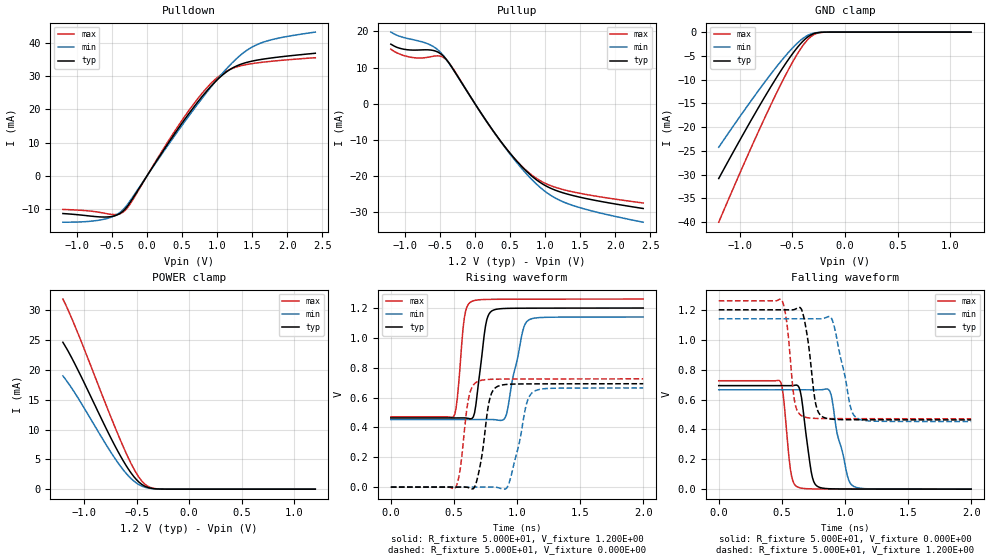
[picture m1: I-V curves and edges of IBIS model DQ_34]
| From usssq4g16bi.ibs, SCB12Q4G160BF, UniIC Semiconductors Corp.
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|   Model DQ_34
[Model] DQ_34
Model_type I/O
Polarity   Non-Inverting
Enable   Active-High
Vinl =  8.300E-01
Vinh =  9.700E-01
Vmeas =  8.400E-01
Rref =  5.000E+01
Vref =  1.200E+00
C_comp   7.488E-13   7.319E-13   7.703E-13
C_comp_pullup   2.702E-13   2.654E-13   2.792E-13
C_comp_pulldown   4.786E-13   4.665E-13   4.911E-13
[Model Spec]
Vinh   9.700E-01   9.250E-01   1.015E+00
Vinl   8.300E-01   7.850E-01   8.750E-01
Vmeas   8.400E-01   7.980E-01   8.820E-01
Vref   1.200E+00   1.140E+00   1.260E+00
Rref   5.000E+01   5.000E+01   5.000E+01
[Temperature Range]   45.000   95.000   -40.000
[Voltage Range]   1.200E+00   1.140E+00   1.260E+00
[C Comp Corner]
C_comp_pullup   2.702E-13   2.654E-13   2.792E-13
C_comp_pulldown   4.786E-13   4.665E-13   4.911E-13
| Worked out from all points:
|   slope of the pulldown table from 0 to 0.18 V, typ, clamps not added: 30.5 ohm
|   slope of the pullup table from 0 to 0.18 V, typ, clamps not added: 34 ohm
|   GND clamp passes 1 mA (typ) near -0.35 V on its own axis
|   POWER clamp passes 1 mA (typ) near -0.46 V on its own axis
|   rising waveform, R_fixture 5.000E+01, V_fixture 1.200E+00: 20-80 % time 63.1ps typ, 95.3ps min, 47.4ps max; typ from 0.463 V to 1.2 V
|   rising waveform, R_fixture 5.000E+01, V_fixture 0.000E+00: 20-80 % time 68.5ps typ, 98.1ps min, 59ps max; typ from 0 V to 0.692 V
|   falling waveform, R_fixture 5.000E+01, V_fixture 0.000E+00: 20-80 % time 63.4ps typ, 97.5ps min, 48.8ps max; typ from 0.693 V to 0 V
|   falling waveform, R_fixture 5.000E+01, V_fixture 1.200E+00: 20-80 % time 64ps typ, 97.1ps min, 53.2ps max; typ from 1.2 V to 0.464 V
[Pulldown]
|Voltage   I(typ)   I(min)   I(max)
-1.2V     -11.33mA   -13.92mA   -10.1mA
-608mV    -12.38mA   -13.02mA   -11.23mA
-423mV    -11.72mA   -11.54mA   -11.58mA
-312mV    -9.977mA   -9.474mA   -10.38mA
280mV     9.088mA    8.608mA    9.642mA
576mV     18.06mA    17.37mA    18.99mA
872mV     25.96mA    25.61mA    26.85mA
1.094V    30.57mA    31.21mA    30.93mA
1.353V    33.61mA    36.57mA    33.11mA
1.575V    34.75mA    39.45mA    33.92mA
1.871V    35.64mA    41.31mA    34.58mA
2.4V      36.79mA    43.15mA    35.45mA
[Pullup]
|Voltage   I(typ)   I(min)   I(max)
-1.2V     16.48mA    19.82mA    15.11mA
-930mV    14.87mA    17.92mA    12.91mA
-634mV    14.86mA    16.24mA    12.99mA
-523mV    14.23mA    14.8mA     13.24mA
-412mV    12.34mA    12.36mA    12.24mA
143mV     -4.23mA    -4.213mA   -4.297mA
439mV     -12.21mA   -12.36mA   -12.27mA
735mV     -18.71mA   -19.42mA   -18.52mA
994mV     -22.56mA   -24.18mA   -21.97mA
1.179V    -24.18mA   -26.46mA   -23.34mA
1.438V    -25.62mA   -28.43mA   -24.58mA
2.4V      -29.01mA   -32.8mA    -27.49mA
[GND_clamp]
|Voltage   I(typ)   I(min)   I(max)
-1.2V     -30.84mA   -24.25mA   -40.04mA
-875mV    -17.92mA   -13.94mA   -23.52mA
-750mV    -13.19mA   -10.17mA   -17.47mA
-625mV    -8.699mA   -6.602mA   -11.7mA
-525mV    -5.384mA   -3.989mA   -7.412mA
-450mV    -3.179mA   -2.281mA   -4.518mA
-375mV    -1.408mA   -958.6uA   -2.123mA
-325mV    -614.2uA   -404.9uA   -980.6uA
-250mV    -97.6uA    -67.88uA   -160.7uA
-175mV    -8.82uA    -7.635uA   -12.18uA
1.2V      0A         0A         0A
[POWER_clamp]
|Voltage   I(typ)   I(min)   I(max)
-1.2V     24.65mA    19.01mA    31.9mA
-1.15V    23.15mA    17.82mA    30.04mA
-1.075V   20.62mA    15.83mA    26.93mA
-775mV    9.691mA    7.064mA    13.48mA
-625mV    4.722mA    3.212mA    7.078mA
-550mV    2.672mA    1.744mA    4.238mA
-500mV    1.586mA    1.017mA    2.629mA
-450mV    802uA      518.6uA    1.374mA
-400mV    337uA      230.9uA    568.8uA
-350mV    119.1uA    91.13uA    183.1uA
-250mV    9.454uA    10.16uA    10.01uA
1.2V      0A         0A         2.743nA
[Ramp]
| variable   typ   min   max
dV/dt_r   4.155E-01/6.895E-11   3.985E-01/9.896E-11   4.351E-01/6.008E-11
dV/dt_f   4.419E-01/6.416E-11   4.124E-01/9.723E-11   4.735E-01/5.414E-11
R_load = 5.000E+01
[Rising Waveform]
R_fixture= 5.000E+01
V_fixture= 1.200E+00
V_fixture_min= 1.140E+00
V_fixture_max= 1.260E+00
|time   V(typ)   V(min)   V(max)
0s        463.1mV    452.2mV    470.6mV
497ps     463mV      452.2mV    471.4mV
527ps     463.1mV    452.2mV    597.2mV
582ps     463.2mV    452.2mV    1.131V
644ps     460.1mV    452.2mV    1.245V
751ps     1.083V     452.3mV    1.257V
799ps     1.179V     452.3mV    1.258V
916ps     1.197V     487mV      1.259V
1.087ns   1.199V     1.116V     1.259V
2ns       1.2V       1.139V     1.26V
[Rising Waveform]
R_fixture= 5.000E+01
V_fixture= 0.000E+00
V_fixture_min= 0.000E+00
V_fixture_max= 0.000E+00
|time   V(typ)   V(min)   V(max)
0s        323.6nV    813.2nV    147.7nV
507ps     -137.7uV   1.048uV    -10.42mV
547ps     -14.19uV   2.927uV    104.6mV
622ps     -5.832mV   13.42uV    617.4mV
691ps     76.19mV    -95.66uV   708.3mV
779ps     572.8mV    289.4uV    721.5mV
838ps     670.9mV    -1.692mV   723mV
937ps     688.9mV    27.35mV    723.8mV
1.13ns    691.4mV    638.7mV    724.2mV
2ns       692.4mV    664.1mV    725.1mV
[Falling Waveform]
R_fixture= 5.000E+01
V_fixture= 0.000E+00
V_fixture_min= 0.000E+00
V_fixture_max= 0.000E+00
|time   V(typ)   V(min)   V(max)
0s        692.9mV    664.8mV    725.4mV
482ps     692.9mV    664.8mV    726.4mV
512ps     692.8mV    664.8mV    623.2mV
568ps     692.6mV    664.8mV    131.8mV
626ps     692.9mV    664.7mV    14.48mV
732ps     120.7mV    664.5mV    2.328mV
782ps     19.04mV    664.6mV    1.644mV
889ps     2.7mV      635.6mV    1.21mV
1.061ns   1.179mV    23.07mV    926.9uV
2ns       338.2uV    502.6uV    249.6uV
[Falling Waveform]
R_fixture= 5.000E+01
V_fixture= 1.200E+00
V_fixture_min= 1.140E+00
V_fixture_max= 1.260E+00
|time   V(typ)   V(min)   V(max)
0s        1.2V       1.14V      1.26V
501ps     1.2V       1.14V      1.263V
538ps     1.2V       1.14V      1.124V
598ps     1.202V     1.14V      603.7mV
666ps     1.178V     1.14V      487.1mV
762ps     599.3mV    1.14V      473.9mV
820ps     485.8mV    1.14V      472.6mV
900ps     468.2mV    1.131V     472.1mV
1.094ns   464.5mV    476.6mV    471.6mV
2ns       463.5mV    452.7mV    470.9mV
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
